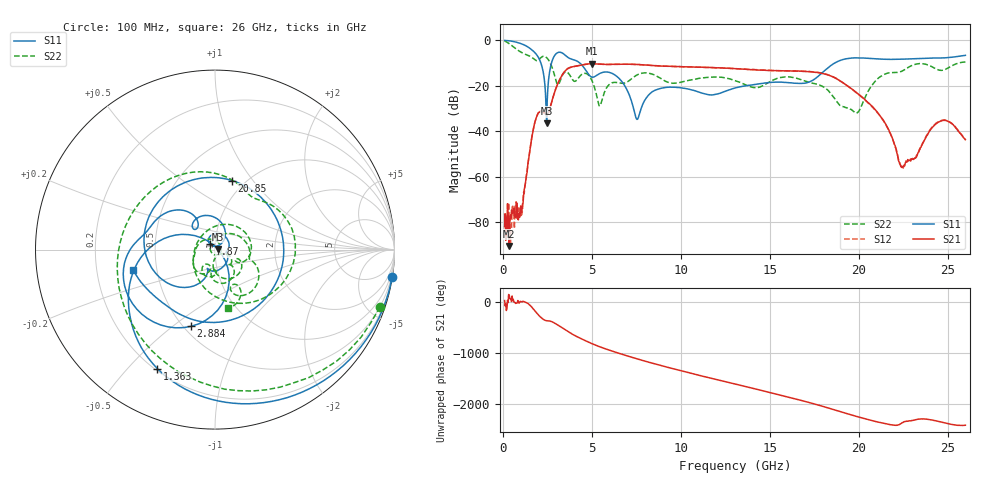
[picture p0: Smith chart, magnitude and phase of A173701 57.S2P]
!  2-Port S-parameters saved by WinCal
! VAR MeasName=S-Parameters (CALIBRATED_DATA) read from VNA (N5245A)
! VAR MeasDate=2017-6-7 10:32:12
! VAR NAME=A173701 57
! VAR FILENAME=A173701 57.S2P
! VAR DATE=2017-6-7 10:32:12
! VAR PHYS_PORTS=1,2
# Hz S DB R 50
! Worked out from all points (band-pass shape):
!   801 points, 100 MHz to 26 GHz, reference 50 ohm
!   highest |S21| = -10.28 dB at 5.021 GHz (marker M1); lowest = -90.5 dB at 359 MHz (marker M2)
!   |S21| within 3 dB of the highest: 3.522 GHz to 14.96 GHz (11.44 GHz wide, 124 % of centre); 14.96 GHz to 15.04 GHz (82.49 MHz wide, 0.55 % of centre)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
!   lowest |S11| = -36.5 dB at 2.463 GHz (marker M3), VSWR 1.03, Z = 51.5 + j0.31 ohm
!   |S11| at or under -10 dB: 2.142 GHz to 2.733 GHz (591.7 MHz wide, 24.3 % of centre); 4.333 GHz to 18.64 GHz (14.31 GHz wide, 125 % of centre)
!   |S22| runs from -32.0 to -0.2 dB; largest |S21 - S12| = 0.0036
!   S11 on the Smith chart (normalised r, x): 100 MHz: 0, -13; 1.363 GHz: 0.21, -0.61; 2.884 GHz: 0.54, -0.58; 7.87 GHz: 0.95, +0.06; 20.85 GHz: 0.87, +0.80; 26 GHz: 0.37, -0.11
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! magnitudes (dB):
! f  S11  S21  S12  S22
! 100 MHz  0.0  -82.0  -76.1  -0.2
! 359 MHz  -0.2  -90.5  -84.7  -1.4
! 974.1 MHz  -1.3  -76.7  -72.9  -5.0
! 1.363 GHz  -2.7  -58.3  -57.2  -6.4
! 1.881 GHz  -6.1  -34.0  -34.0  -8.9
! 2.463 GHz  -36.5  -32.8  -32.8  -7.6
! 2.884 GHz  -7.0  -23.4  -23.3  -14.7
! 4.438 GHz  -10.8  -10.8  -10.8  -15.0
! 5.021 GHz  -16.2  -10.3  -10.3  -17.9
! 5.474 GHz  -14.5  -10.4  -10.5  -28.7
! 6.64 GHz  -17.6  -10.5  -10.5  -18.8
! 7.514 GHz  -34.6  -10.6  -10.6  -15.3
! 7.87 GHz  -28.0  -10.8  -10.8  -14.4
! 8.744 GHz  -21.4  -11.2  -11.2  -16.2
! 13.05 GHz  -21.0  -12.4  -12.4  -17.7
! 17.39 GHz  -17.7  -13.9  -13.8  -18.8
! 19.85 GHz  -7.7  -22.8  -22.9  -32.0
! 20.85 GHz  -8.0  -29.8  -30.0  -18.7
! 21.69 GHz  -8.3  -39.4  -39.7  -14.3
! 22.47 GHz  -8.2  -55.8  -56.0  -13.4
! 24.54 GHz  -7.7  -35.8  -35.6  -13.1
! 26 GHz  -6.6  -43.7  -43.9  -9.5
